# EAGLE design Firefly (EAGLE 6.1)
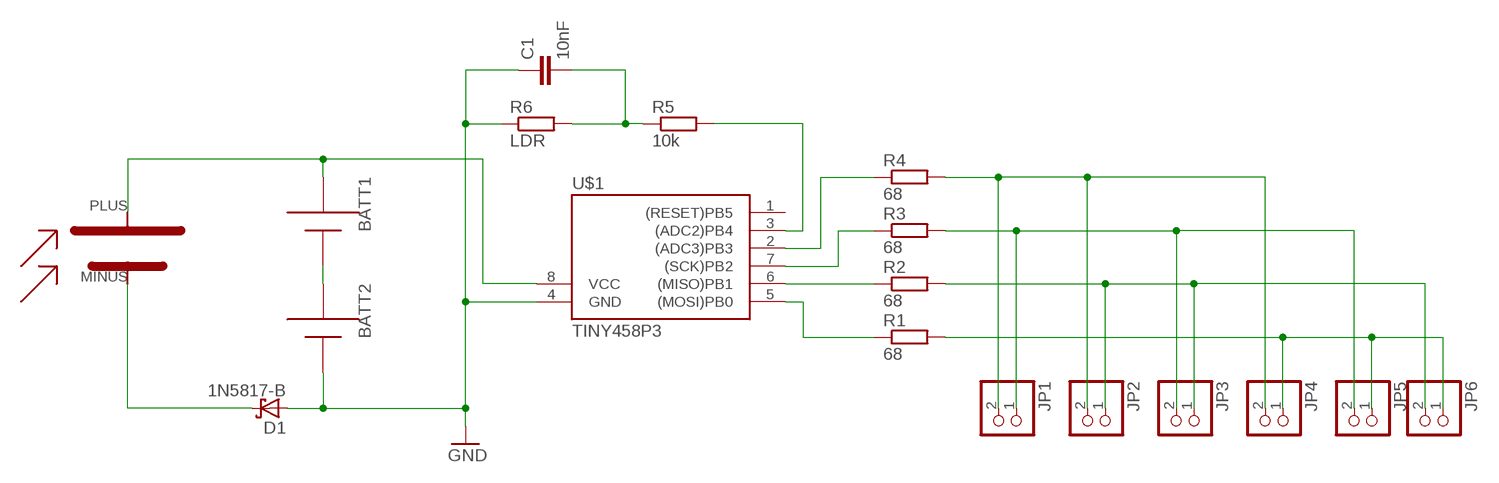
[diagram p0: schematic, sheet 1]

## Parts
BATT1  AAA  [12BH412]
BATT2  AAA  [12BH412]
C1  10nF  C-EU025-025X050  [C025-025X050]
D1  1N5817-B  [DO41-7.6]
JP1  PINHD-1X2  [1X02]
JP2  PINHD-1X2  [1X02]
JP3  PINHD-1X2  [1X02]
JP4  PINHD-1X2  [1X02]
JP5  PINHD-1X2  [1X02]
JP6  PINHD-1X2  [1X02]
R1  68  R-EU_0207/10  [0207/10]
R2  68  R-EU_0207/12  [0207/12]
R3  68  R-EU_0207/10  [0207/10]
R4  68  R-EU_0207/10  [0207/10]
R5  10k  R-EU_0207/10  [0207/10]
R6  LDR  R-EU_0207/10  [0207/10]
U$1  TINY458P3  [DIL08]
U$2  SOLARCELL4V35MACONRAD  [SOLARCELL35X39]

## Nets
GND: BATT2.- C1.1 D1.A R6.1 U$1.4(GND)
N$1: R1.1 U$1.5((MOSI)PB0)
N$2: R2.1 U$1.6((MISO)PB1)
N$3: R3.1 U$1.7((SCK)PB2)
N$4: R4.1 U$1.2((ADC3)PB3)
N$5: JP1.2 JP2.2 JP4.2 R4.2
N$6: BATT1.- BATT2.+
N$7: JP2.1 JP3.1 JP6.2 R2.2
N$8: JP1.1 JP3.2 JP5.2 R3.2
N$10: JP4.1 JP5.1 JP6.1 R1.2
N$11: BATT1.+ U$1.8(VCC) U$2.PLUS
N$12: D1.C U$2.MINUS
N$13: R5.2 U$1.3((ADC2)PB4)
N$14: C1.2 R5.1 R6.2
Unconnected: U$1.1((RESET)PB5)

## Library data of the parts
BATT1 BATT2 = adafruit:AAA: AAA PC pin holder
C1 = resistor:C-EU: CAPACITOR, European symbol
D1 = diode:1N581*: 1.0A SCHOTTKY BARRIER RECTIFIER
JP1-JP6 = pinhead:PINHD-1X2: PIN HEADER
R1-R6 = resistor:R-EU_: RESISTOR, European symbol
U$1 = firefly:TINY45*
U$2 = firefly:SOLARCELL4V35MACONRAD: Conrad Miniatur-Solarzellen Monokristallin Nennspannung 4 V Nennstrom 35 mA

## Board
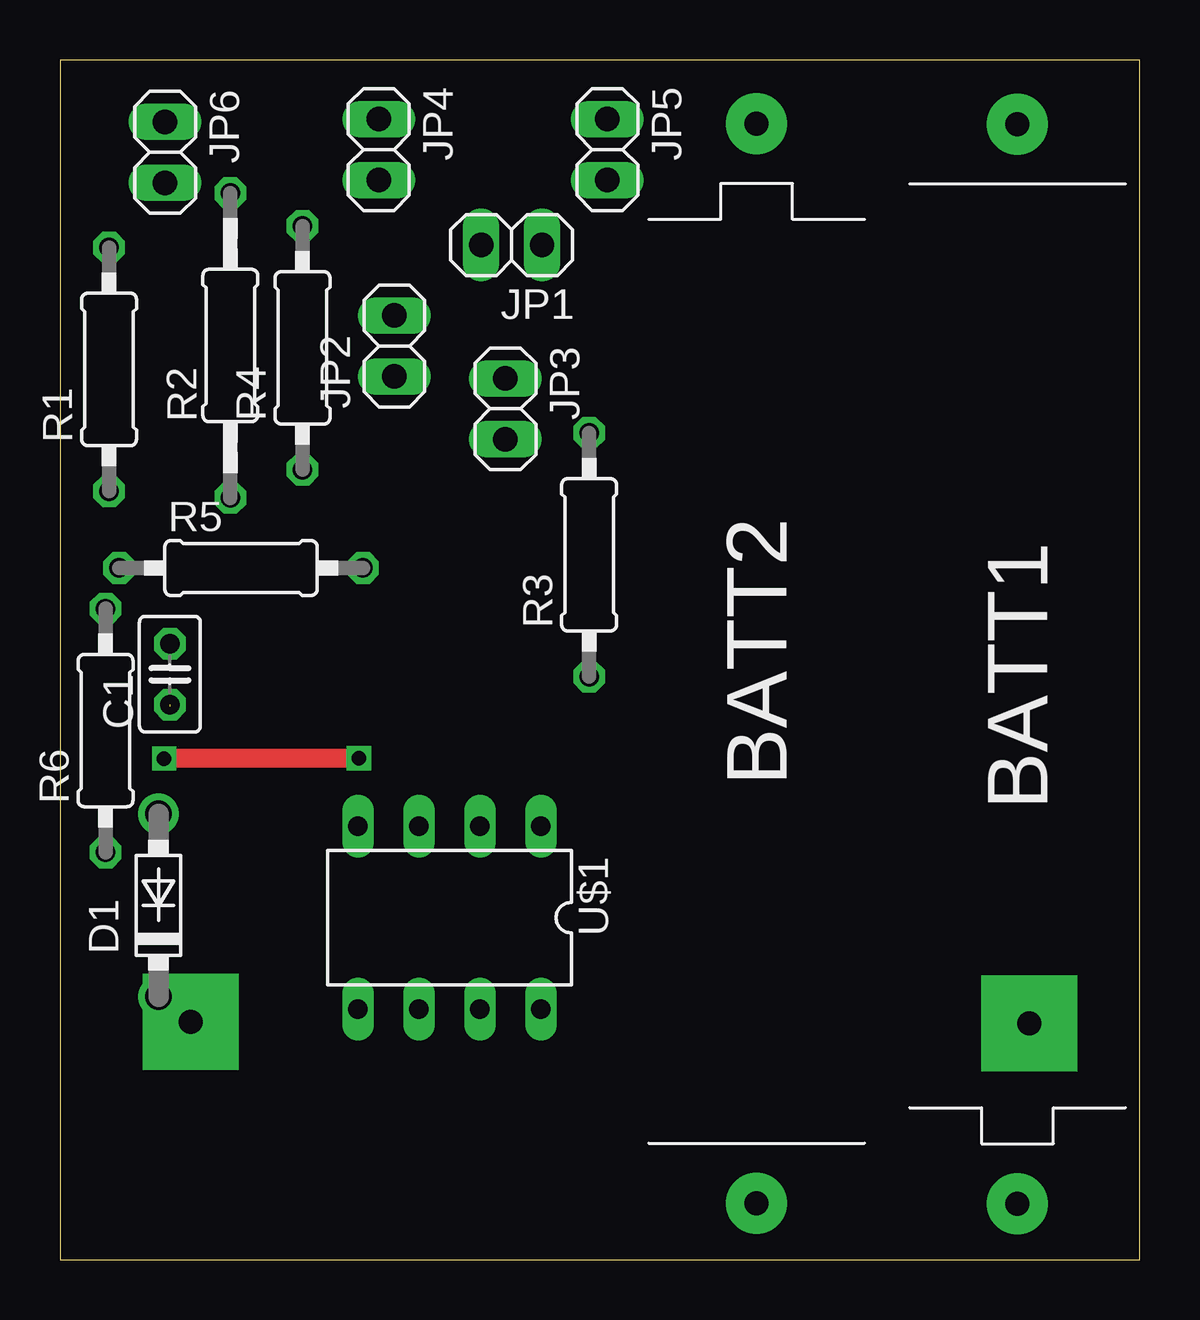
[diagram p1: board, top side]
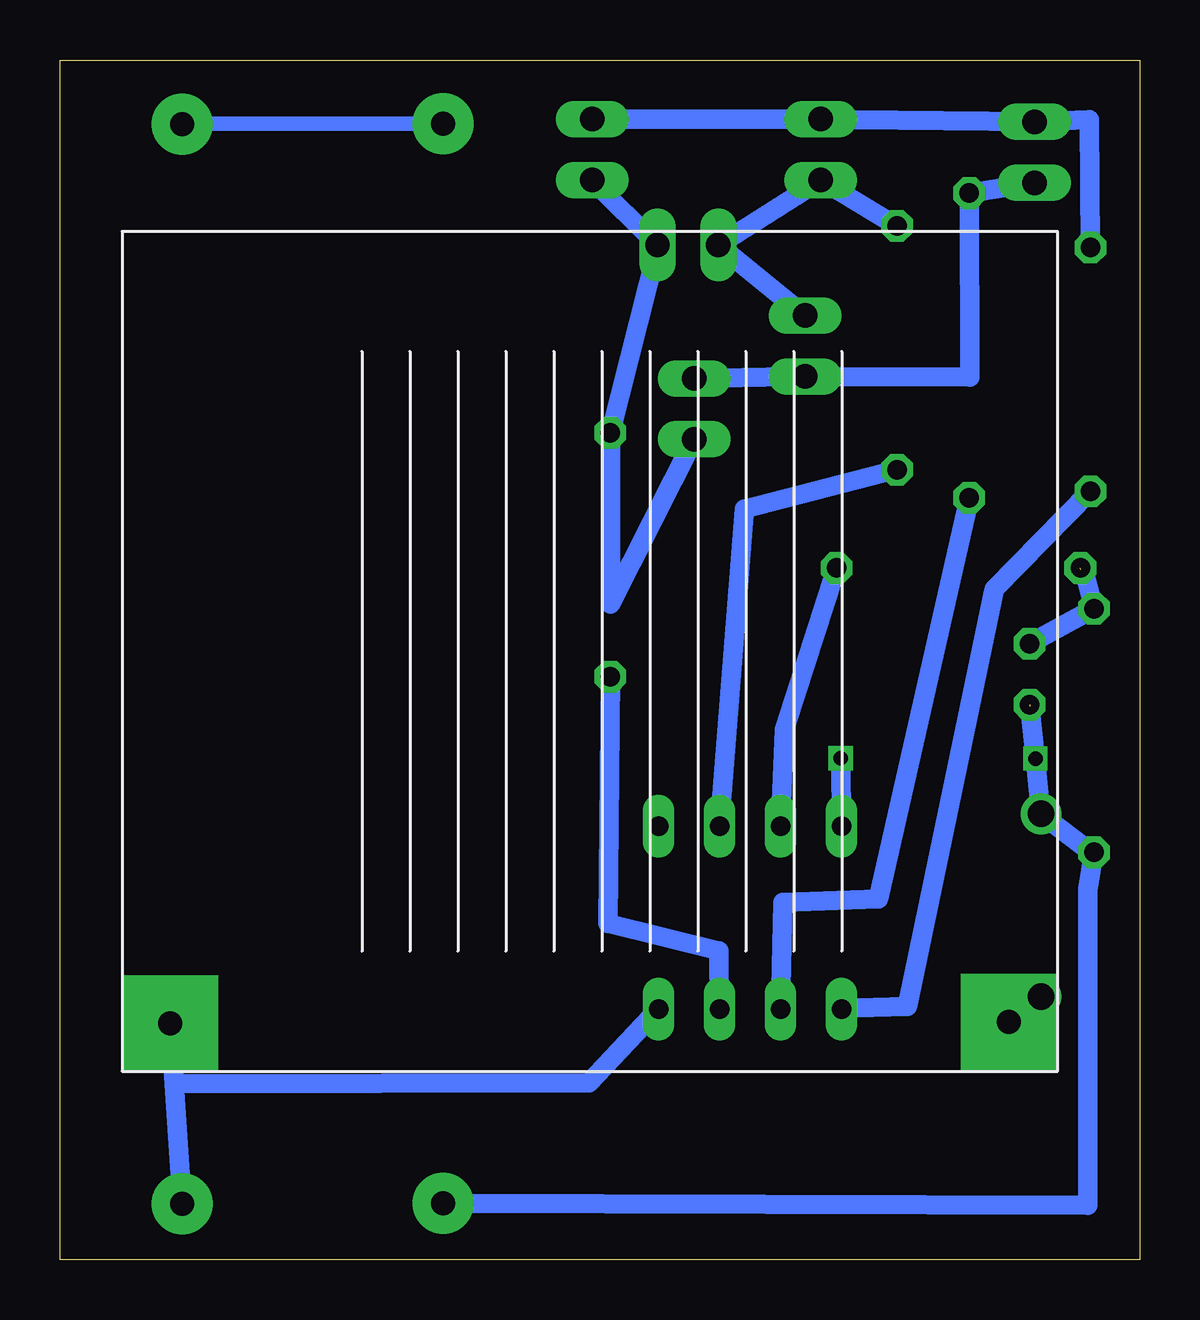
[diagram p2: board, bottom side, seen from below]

Size 45 x 50 mm. Coordinates in mm from the lower left corner, seen from the top.
Outline: 0,0 45,0 45,50 0,50 0,0
Copper layers (1*16): Top 0.035mm / dielectric 1.5mm / Bottom 0.035mm
Design rules: minimum track width 10mil, minimum drill 24mil, track to track 8mil, track to pad 8mil, pad to pad 8mil, via to via 8mil, smd to smd 8mil, copper to edge 40mil, drill to drill 8mil, minimum pad ring 10mil, minimum via ring 8mil, stop-mask expansion 4mil, vias tented up to drill 0mil, thermal gap 10mil

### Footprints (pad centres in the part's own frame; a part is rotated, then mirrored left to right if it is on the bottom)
12BH412 = drill 1 pad 2.54: + 22.5,0; - -22.5,0
C025-025X050 = drill 0.813 octagon: 1 -1.27,0; 2 1.27,0
DO41-7.6 = drill 1.1 pad 1.7: A 3.81,0; C -3.81,0
1X02 = drill 1.016 long: 1 -1.27,0; 2 1.27,0
0207/10 = drill 0.813 octagon: 1 -5.08,0; 2 5.08,0
0207/12 = drill 0.813 octagon: 1 -6.35,0; 2 6.35,0
DIL08 = drill 0.813 long: 1 -3.81,-3.81; 2 -1.27,-3.81; 3 1.27,-3.81; 4 3.81,-3.81; 5 3.81,3.81; 6 1.27,3.81; 7 -1.27,3.81; 8 -3.81,3.81
SOLARCELL35X39 = drill 1 pad 4 square: MINUS 36.96,2.07; PLUS 2,2

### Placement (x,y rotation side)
BATT1  39.91,24.83 270 top
BATT2  29.04,24.85 90 top
C1  4.58,24.4 90 top
D1  4.11,14.77 90 top
JP1  18.83,42.29 180 top
JP2  13.94,38.08 90 top
JP3  18.57,35.46 270 top
JP4  13.29,46.27 270 top
JP5  22.82,46.27 270 top
JP6  4.38,46.15 270 top
R1  2.04,37.1 90 top
R2  7.1,38.1 90 top
R3  22.06,29.38 90 top
R4  10.11,38 90 top
R5  7.55,28.82 0 top
R6  1.9,22.05 90 top
U$1  16.23,14.25 180 top
U$2  42.42,7.84 0 bottom

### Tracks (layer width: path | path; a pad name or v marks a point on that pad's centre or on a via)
GND  (via drill 0.6)  (1 unrouted)
  Top 0.813: v4.34,20.88 v12.46,20.9
  Bottom 0.813: BATT2.- 2.16,2.25 2.16,15.43 R6.1 2.02,16.97 D1.A v4.34,20.88 4.58,23.06 | U$1.4 v12.46,20.9
N$1
  Bottom 0.813: R1.1 6.06,27.95 9.67,10.54 12.48,10.48 | 12.48,10.48 12.63,10.47 | U$1.5 12.48,10.48
N$2
  Bottom 0.813: U$1.6 14.86,14.88 10.9,15.02 R2.1
N$3
  Bottom 0.813: U$1.7 17.53,12.86 22.15,14.01 R3.1
N$4
  Bottom 0.813: U$1.2 16.46,31.29 R4.1
N$5
  Bottom 0.813: R4.2 JP4.2 JP1.2 JP2.2
N$6
  Bottom 0.406: 39.91,47.35 BATT1.-
  Bottom 0.61: BATT2.+ 39.91,47.35
N$7
  Bottom 0.813: JP3.1 14.58,36.8 | 14.58,36.8 JP2.1 | JP6.2 R2.2 7.07,36.79 14.58,36.8
N$8
  Bottom 0.813: JP5.2 JP1.1 20.1,42.17 R3.2 22.05,27.32 JP3.2
N$10
  Bottom 0.813: JP4.1 13.85,47.54 | 13.85,47.54 JP5.1 | 13.85,47.54 JP6.1 2.09,47.51 R1.2
N$11
  Bottom 0.813: BATT1.+ 40.25,7.33 | 40.25,7.33 U$2.PLUS | U$1.8 22.94,7.37 40.25,7.33
N$12
  Bottom 0.813: U$2.MINUS D1.C
N$13
  Bottom 0.813: U$1.3 14.79,22.1 R5.2
N$14  (1 unrouted)
  Bottom 0.813: C1.2 R6.2 2.35,28.92 2.46,28.77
